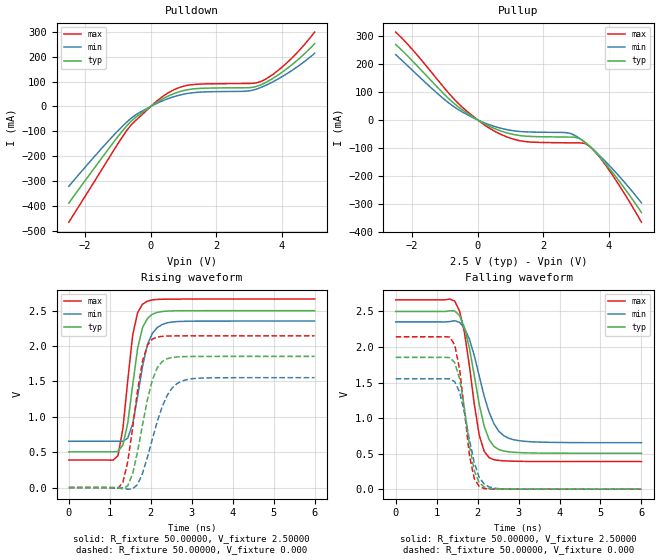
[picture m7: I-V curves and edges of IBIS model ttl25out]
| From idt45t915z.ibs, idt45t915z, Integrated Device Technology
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|   Model ttl25out
[Model]   ttl25out
Model_type   Output
Polarity   Non-Inverting
Vmeas =  1.25000V
C_comp   5.00000pF   5.00000pF   5.00000pF
[Temperature Range]   45.00000   0.14000k   -30.00000
[Voltage Range]   2.50000V   2.30000V   2.70000V
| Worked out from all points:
|   slope of the pulldown table from 0 to 0.375 V, typ, clamps not added: 12.1 ohm
|   slope of the pullup table from 0 to 0.375 V, typ, clamps not added: 15.8 ohm
|   rising waveform, R_fixture 50.00000, V_fixture 2.50000: 20-80 % time 299ps typ, 329ps min, 257ps max; typ from 0.505 V to 2.5 V
|   rising waveform, R_fixture 50.00000, V_fixture 0.000: 20-80 % time 397ps typ, 498ps min, 324ps max; typ from 0 V to 1.85 V
|   falling waveform, R_fixture 50.00000, V_fixture 2.50000: 20-80 % time 402ps typ, 495ps min, 340ps max; typ from 2.5 V to 0.505 V
|   falling waveform, R_fixture 50.00000, V_fixture 0.000: 20-80 % time 302ps typ, 343ps min, 267ps max; typ from 1.85 V to 0 V
[Pulldown]
| voltage   I(typ)   I(min)   I(max)
-2.5V     -387.1mA   -320.1mA   -464mA
-1.3V     -172.3mA   -139.4mA   -211.9mA
-700mV    -73.11mA   -58.92mA   -90.86mA
-400mV    -37.65mA   -28.88mA   -48.96mA
300mV     25.63mA    19.24mA    33.79mA
700mV     51.07mA    38.83mA    66.42mA
1.1V      66.37mA    51.46mA    84.22mA
2.9V      74.99mA    61.06mA    92.02mA
3.4V      89.1mA     78.19mA    102.5mA
4.1V      145.9mA    126.7mA    168.2mA
4.5V      188.2mA    161.4mA    220mA
5V        251.4mA    212.9mA    298.1mA
[Pullup]
| voltage   I(typ)   I(min)   I(max)
-2.5V     269.9mA    233.5mA    314.3mA
-800mV    67.39mA    53.61mA    84.83mA
-300mV    22.62mA    17.64mA    28.64mA
400mV     -25.11mA   -19.06mA   -32.59mA
900mV     -46.72mA   -35.05mA   -61.28mA
1.4V      -57.66mA   -42.47mA   -76.9mA
2.8V      -61.54mA   -47.61mA   -82.16mA
3.1V      -66.62mA   -65.23mA   -82.46mA
3.4V      -92.17mA   -92.61mA   -92.89mA
3.7V      -128.7mA   -125.1mA   -129.7mA
4.1V      -185.6mA   -173.4mA   -194.7mA
5V        -331.7mA   -297.2mA   -366.3mA
[Ramp]
| variable   typ   min   max
dV/dt_r   1.11240/0.40582n   0.93180/0.51868n   1.28700/0.32381n
dV/dt_f   1.19718/0.40734n   1.02540/0.48502n   1.36524/0.35328n
R_load = 50.00000
[Rising Waveform]
R_fixture = 50.00000
V_fixture = 2.50000
C_fixture = 0.000F
R_dut = 6.00000m
L_dut = 3.00000nH
C_dut = 0.20000pF
| time   V(typ)   V(min)   V(max)
0s        504.9mV    653.9mV    388.5mV
1.2ns     511.8mV    654mV      449.4mV
1.32ns    600mV      653.5mV    831mV
1.44ns    916.8mV    698.2mV    1.52V
1.56ns    1.452V     905.6mV    2.158V
1.68ns    1.968V     1.29V      2.473V
1.8ns     2.263V     1.714V     2.592V
2.04ns    2.45V      2.18V      2.652V
2.4ns     2.494V     2.328V     2.663V
6ns       2.5V       2.353V     2.664V
[Rising Waveform]
R_fixture = 50.00000
V_fixture = 0.000
C_fixture = 0.000F
R_dut = 6.00000m
L_dut = 3.00000nH
C_dut = 0.20000pF
| time   V(typ)   V(min)   V(max)
0s        0V         0V         0V
1.2ns     -7.736mV   74.99uV    -11.29mV
1.32ns    -16.35mV   -5.463mV   72.34mV
1.44ns    25.8mV     -22.87mV   368.6mV
1.56ns    199.1mV    -17.97mV   853mV
1.8ns     889.2mV    201.3mV    1.786V
2.04ns    1.522V     686.6mV    2.099V
2.4ns     1.821V     1.301V     2.142V
2.76ns    1.85V      1.506V     2.144V
6ns       1.854V     1.553V     2.144V
[Falling Waveform]
R_fixture = 50.00000
V_fixture = 2.50000
C_fixture = 0.000F
R_dut = 6.00000m
L_dut = 3.00000nH
C_dut = 0.20000pF
| time   V(typ)   V(min)   V(max)
0s        2.5V       2.353V     2.664V
1.44ns    2.508V     2.37V      2.647V
1.56ns    2.442V     2.346V     2.506V
1.68ns    2.272V     2.263V     2.199V
1.8ns     1.984V     2.11V      1.734V
2.04ns    1.192V     1.591V     758.1mV
2.28ns    697.5mV    1.083V     443mV
2.52ns    556.5mV    813.2mV    404mV
2.88ns    519mV      695.7mV    393.1mV
6ns       504.9mV    654mV      388.5mV
[Falling Waveform]
R_fixture = 50.00000
V_fixture = 0.000
C_fixture = 0.000F
R_dut = 6.00000m
L_dut = 3.00000nH
C_dut = 0.20000pF
| time   V(typ)   V(min)   V(max)
0s        1.854V     1.553V     2.144V
1.32ns    1.851V     1.552V     2.14V
1.44ns    1.783V     1.512V     2.031V
1.56ns    1.554V     1.367V     1.687V
1.8ns     618.1mV    696.3mV    476.7mV
1.92ns    255.7mV    369mV      145.9mV
2.04ns    90.47mV    165.6mV    37.04mV
2.28ns    10.07mV    32.31mV    3.092mV
2.52ns    2.521mV    7.211mV    1.099mV
6ns       941.7nV    3.235uV    0V
